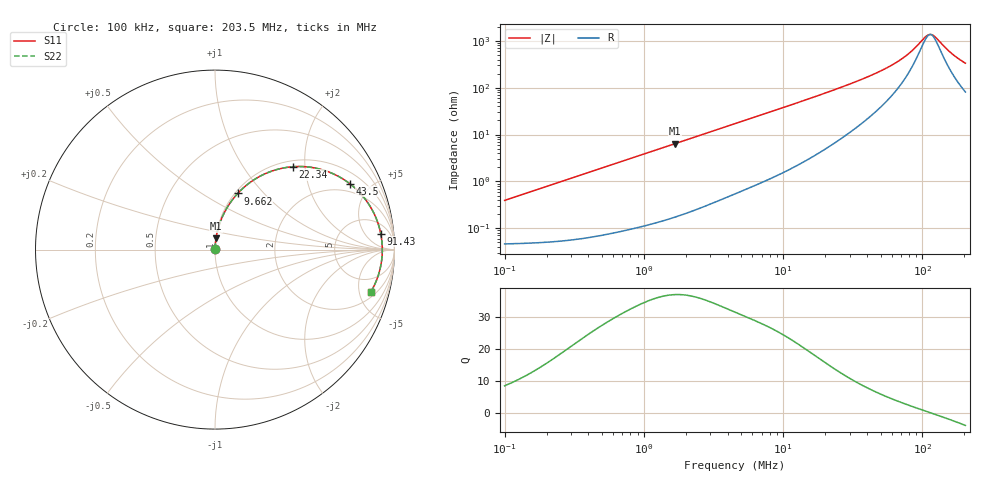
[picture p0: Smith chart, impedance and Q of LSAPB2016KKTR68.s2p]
! LSAPB2016KKTR68  S-PARAMETER MODEL  ( General Type )
! Model Generated by TAIYO YUDEN Corporation (http://www.ty-top.com)
! Version 2.0
! TAIYO YUDEN Control No. 20210629
! Copyright(c) 2015 TAIYO YUDEN CO.,LTD. All Rights Reserved.
! Product Description (link to TY-COMPAS)
! https://ds.yuden.co.jp/TYCOMPAS/or/detail?pn=LSAPB2016KKTR68M&u=M
! Products Name : Inductors
! Characteristics :
!  Inductance : 0.68 uH , SRF(min) : -Hz , DC Resistance(max) : 0.05 Ohm
!  Rated Current : Saturation :3200 mA , Temp Rise : 2700 mA (40 degC)
!  Case Size : 2.0 x 1.6 / 0.079 x 0.063 [mm/inch] , Thickness : 1 / 0.039 [mm/inch]
!  (Conditions: Temperature = 25 degC , DC Bias Current/Voltage = 0A / 0V)
! External Node Assignments :
!  1  o---GGG---o  2
! GND o---------o GND
! Frequency Range : 0.1MHz  -  203.457813MHz  [ 402 STEP ]
# MHz S RI R 50
! Freq[MHz].  S11 Real  S11 Imag  S21 Real  S21 Imag  S12 Real  S12 Imag  S22 Real  S22 Imag
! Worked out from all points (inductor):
!   401 points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, 100 kHz to 203.5 MHz, reference 50 ohm
!   read as one part in series: L = 621 nH near 103.9 kHz
!   highest Q = 37.1 at 1.675 MHz (marker M1), where L = 609 nH
!   self-resonance near 113.8 MHz
!   S11 on the Smith chart (normalised r, x): 100 kHz: 1.00, +0.01; 9.662 MHz: 1.03, +0.73; 22.34 MHz: 1.12, +1.72; 43.5 MHz: 1.53, +3.72; 91.43 MHz: 10, +13; 203.5 MHz: 2.62, -6.49
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0.1  0.000477 0.0039  0.9995 -0.0039  0.9995 -0.0039  0.000477 0.0039
0.358236  0.000793 0.0139  0.9992 -0.0139  0.9992 -0.0139  0.000793 0.0139
1.283332  0.00376 0.049  0.9962 -0.049  0.9962 -0.049  0.00376 0.049
1.675466  0.0058 0.0636  0.9942 -0.0636  0.9942 -0.0636  0.0058 0.0636
4.51063  0.0332 0.1641  0.9668 -0.1641  0.9668 -0.1641  0.0332 0.1641
6.858092  0.0701 0.2381  0.9299 -0.2381  0.9299 -0.2381  0.0701 0.2381
9.662391  0.1267 0.3132  0.8733 -0.3132  0.8733 -0.3132  0.1267 0.3132
12.61482  0.196 0.3747  0.804 -0.3747  0.804 -0.3747  0.196 0.3747
16.15871  0.2845 0.425  0.7155 -0.425  0.7155 -0.425  0.2845 0.425
22.33659  0.432 0.4617  0.568 -0.4617  0.568 -0.4617  0.432 0.4617
30.87642  0.5955 0.4454  0.4045 -0.4454  0.4045 -0.4454  0.5955 0.4454
43.50191  0.7501 0.3679  0.2499 -0.3679  0.2499 -0.3679  0.7501 0.3679
57.88634  0.8447 0.2706  0.1553 -0.2706  0.1553 -0.2706  0.8447 0.2706
74.14835  0.8979 0.1745  0.1021 -0.1745  0.1021 -0.1745  0.8979 0.1745
91.42912  0.9234 0.0897  0.0766 -0.0897  0.0766 -0.0897  0.9234 0.0897
106.4766  0.9314 0.0273  0.0686 -0.0273  0.0686 -0.0273  0.9314 0.0273
112.7373  0.9322 0.00391  0.0678 -0.00391  0.0678 -0.00391  0.9322 0.00391
117.1143  0.9321 -0.0117  0.0679 0.0117  0.0679 0.0117  0.9321 -0.0117
124.0005  0.9309 -0.0351  0.0691 0.0351  0.0691 0.0351  0.9309 -0.0351
161.89  0.9096 -0.144  0.0904 0.144  0.0904 0.144  0.9096 -0.144
184.9773  0.8885 -0.1975  0.1115 0.1975  0.1115 0.1975  0.8885 -0.1975
203.4578  0.8689 -0.2348  0.1311 0.2348  0.1311 0.2348  0.8689 -0.2348
